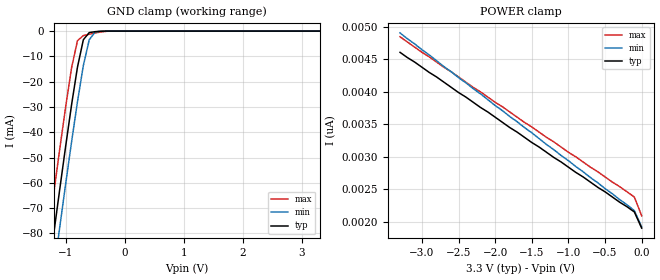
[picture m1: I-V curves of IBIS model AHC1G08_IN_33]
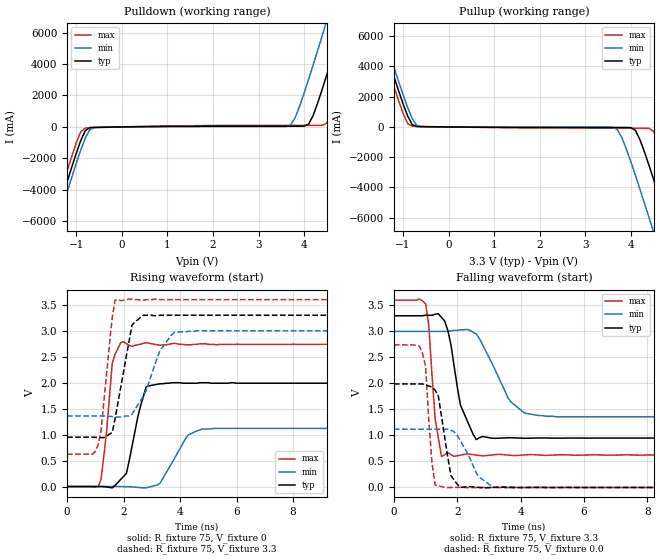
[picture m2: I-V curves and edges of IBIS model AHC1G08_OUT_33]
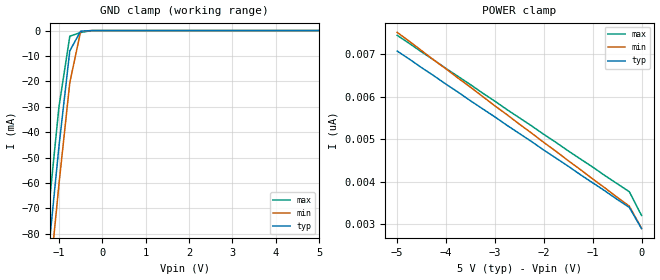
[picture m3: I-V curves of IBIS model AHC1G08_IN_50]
| TEXAS INSTRUMENTS INCORPORATED
| Standard Linear and Logic Group
| IBIS Model of SN74AHC1G08
| SINGLE 2-INPUT POSITIVE-AND GATE
| SOT 5-pin (DCK) and SOT 5-pin (DBV) Package
[IBIS Ver]   3.2
[Comment Char]  |_char
[File Name]   ahc1g08.ibs
[File Rev]   2.0 J_die
[Date]   May 24, 2000
[Source]   Data created from HSPICE simulations at TI-SLL.
[Notes]   The following is an IBIS list for the AHC1G08.
|   Please contact sllibis@ti.com with questions and
|   comments concerning SLL IBIS models.
[Disclaimer] Property of Texas Instruments Incorporated.  Unauthorized
   reproduction and/or distribution is strictly prohibited.
   This product is protected under copyright law.
   Created 2000, (C) Copyright 2000, Texas Instruments Inc.,
   All Rights Reserved.
   UNLESS THERE IS A SIGNED, WRITTEN AGREEMENT TO THE
   CONTRARY, TEXAS INSTRUMENTS () IS PROVIDING THE IBIS
   MODELS  AND WITHOUT ANY WARRANTY, EXPRESSED OR
   IMPLIED.  TI assumes no liability for:
   1) the accuracy of the IBIS models provided to your
   company;
   2) the proper functioning of these IBIS Models in your
   design or for any resulting applications; or
   3) infringement of patents, copyrights or intellectual
   property rights resulting from your use of these IBIS
   models.
   TI provides IBIS Models as a service to our customers.
   You and your company shall not distribute, sell or give
   these models to anyone else without prior written
   permission from TI.
   TI reserves the right to make changes to our products or
   to discontinue any semiconductor product or service
   without notice, and advises our customers to obtain the
   latest version of relevant information to verify, before
   placing orders, that the information being relied on is
   current.
   Please be aware that your receipt and use of the IBIS
   information provided shall serve as acceptance of these
   terms and conditions.  If you do not accept these terms,
   you should return or destroy the IBIS models and any
   other accompanying information immediately.
|   Component AHC1G08_DCK
[Component]   AHC1G08_DCK
[Manufacturer]  Texas Instruments, Inc.
[Package]
|   typ   min   max
R_pkg   0.020   0.017   0.025
L_pkg   0.998nH   0.881nH   1.069nH
C_pkg   0.146pF   0.118pF   0.205pF
[Pin]   signal_name   model_name   R_pin   L_pin   C_pin
1   A   AHC1G08_IN   0.019   1.069nH   0.162pF
2   B   AHC1G08_IN   0.018   0.881nH   0.121pF
3   GND   GND   0.017   1.031nH   0.205pF
4   Y   AHC1G08_OUT   0.020   0.960nH   0.124pF
5   VCC   POWER   0.025   1.049nH   0.118pF
|   Component AHC1G08_DBV
[Component]   AHC1G08_DBV
[Manufacturer]  Texas Instruments, Inc.
[Package]
|   typ   min   max
R_pkg   0.025   0.021   0.029
L_pkg   1.529nH   1.312nH   1.906nH
C_pkg   0.156pF   0.110pF   0.240pF
[Pin]   signal_name   model_name   R_pin   L_pin   C_pin
1   A   AHC1G08_IN   0.021   1.511nH   0.144pF
2   B   AHC1G08_IN   0.023   1.312nH   0.138pF
3   GND   GND   0.029   1.906nH   0.240pF
4   Y   AHC1G08_OUT   0.026   1.541nH   0.150pF
5   VCC   POWER   0.025   1.374nH   0.110pF
[Model Selector]   AHC1G08_IN
AHC1G08_IN_33   3.3-V Vcc Input Model
AHC1G08_IN_50   5.0-V Vcc Input Model
[Model Selector]   AHC1G08_OUT
AHC1G08_OUT_33   3.3-V Vcc Output Model
AHC1G08_OUT_50   5.0-V Vcc Output Model
| Models and submodels in the file (4): AHC1G08_IN_33 (Input), AHC1G08_OUT_33 (Output), AHC1G08_IN_50 (Input), AHC1G08_OUT_50 (Output)
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|   Model AHC1G08_IN_33
[Model]   AHC1G08_IN_33
Model_type  Input
Polarity   Inverting
Vinl = 0.99
Vinh = 2.31
| variable   typ   min   max
C_comp   1.27pf   0.95pf   1.59pf
[Temperature Range]   25   85   -40
[Voltage Range]   3.3   3.0   3.6
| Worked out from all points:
|   GND clamp passes 1 mA (typ) near -0.61 V on its own axis
[GND Clamp]
|   Voltage   I(typ)   I(min)   I(max)
-3.3V     -460mA     -475mA     -445mA
-1.3V     -97.5mA    -113mA     -81.5mA
-1.2V     -79.9mA    -95mA      -63.9mA
-1.1V     -62.6mA    -77.6mA    -46.7mA
-1V       -45.6mA    -60.5mA    -30mA
-900mV    -29.2mA    -43.9mA    -14.6mA
-800mV    -14.3mA    -28mA      -3.81mA
-700mV    -3.42mA    -13.6mA    -1.78mA
-600mV    -581uA     -3.4mA     -1.25mA
-500mV    -233uA     -353uA     -759uA
-400mV    -58.1uA    -21.9uA    -324uA
3.3V      1.9nA      2.34nA     1.69nA
[POWER Clamp]
|   Voltage   I(typ)   I(min)   I(max)
-3.3V     4.61nA     4.91nA     4.85nA
-3V       4.38nA     4.65nA     4.61nA
-100mV    2.15nA     2.17nA     2.38nA
0V        1.9nA      1.92nA     2.09nA
|   Model AHC1G08_OUT_33
[Model]   AHC1G08_OUT_33
Model_type  Output
Polarity   Inverting
Vmeas = 1.65v
Cref = 15pf
| variable   typ   min   max
C_comp   3.12pf   2.34pf   3.90pf
[Temperature Range]   25   85   -40
[Voltage Range]   3.3   3.0   3.6
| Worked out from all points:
|   slope of the pulldown table from 0 to 0.495 V, typ, clamps not added: 26.1 ohm
|   slope of the pullup table from 0 to 0.495 V, typ, clamps not added: 40.3 ohm
|   rising waveform, R_fixture 75, V_fixture 0: 20-80 % time 464ps typ, 702ps min, 278ps max; typ from 0 V to 1.99 V
|   falling waveform, R_fixture 75, V_fixture 3.3: 20-80 % time 446ps typ, 783ps min, 217ps max; typ from 3.3 V to 0.95 V
|   rising waveform, R_fixture 75, V_fixture 3.3: 20-80 % time 470ps typ, 718ps min, 323ps max; typ from 0.95 V to 3.3 V
|   falling waveform, R_fixture 75, V_fixture 0.0: 20-80 % time 308ps typ, 566ps min, 179ps max; typ from 1.99 V to 0 V
[Pulldown]
|   Voltage   I(typ)   I(min)   I(max)
-3.3V     -24A       -24.6A     -23.4A
-1.6V     -7.31A     -7.95A     -6.63A
-1.5V     -6.34A     -6.99A     -5.66A
-1V       -1.69A     -2.33A     -1.02A
-800mV    -234mA     -703mA     -70.7mA
-600mV    -28.4mA    -27.3mA    -48.1mA
3.7V      47.1mA     113mA      100mA
4.1V      173mA      3.03A      101mA
4.4V      2.42A      5.83A      105mA
4.8V      6.17A      9.67A      2.68A
5.2V      10A        13.6A      6.5A
6.6V      23.8A      27.4A      20.3A
[Pullup]
|   Voltage   I(typ)   I(min)   I(max)
-3.3V     23.8A      24.4A      23.2A
-1.6V     7.13A      7.74A      6.5A
-1.5V     6.17A      6.78A      5.53A
-1V       1.53A      2.14A      903mA
-800mV    158mA      559mA      49mA
-600mV    19.5mA     16.8mA     33.4mA
3.7V      -35.9mA    -168mA     -78.9mA
4.1V      -236mA     -3.23A     -83.5mA
4.4V      -2.58A     -6.03A     -95.5mA
4.8V      -6.34A     -9.88A     -2.81A
5.2V      -10.2A     -13.8A     -6.63A
6.6V      -24A       -27.6A     -20.4A
[Ramp]
| variable   typ   min   max
dV/dt_r   1.20E+00/4.62E-10   6.92E-01/6.38E-10   1.65E+00/2.74E-10
dV/dt_f   1.44E+00/4.29E-10   1.01E+00/7.49E-10   1.87E+00/2.29E-10
R_load = 75
[Rising Waveform]
R_fixture = 75
V_fixture = 0
|   Time   V(typ)   V(min)   V(max)
0s        0V         0V         0V
1.2ns     950uV      243uV      135mV
1.4ns     -8.38mV    656uV      1.07V
1.6ns     -25.1mV    1.08mV     2.38V
2ns       195mV      -1.74mV    2.79V
2.8ns     1.92V      -24.1mV    2.77V
3.3ns     1.98V      70.8mV     2.72V
4.3ns     1.99V      1V         2.73V
4.8ns     2V         1.11V      2.75V
25ns      1.99V      1.12V      2.74V
[Falling Waveform]
R_fixture = 75
V_fixture = 3.3
V_fixture_min = 3.0
V_fixture_max = 3.6
|   Time   V(typ)   V(min)   V(max)
0s        3.3V       3V         3.6V
1ns       3.31V      3V         3.53V
1.1ns     3.31V      3V         3.11V
1.3ns     3.33V      3V         1.32V
1.5ns     3.27V      3V         597mV
2.1ns     1.58V      3.03V      622mV
2.6ns     921mV      2.95V      623mV
3.7ns     956mV      1.64V      618mV
4.6ns     952mV      1.38V      624mV
25ns      950mV      1.36V      624mV
[Rising Waveform]
R_fixture = 75
V_fixture = 3.3
V_fixture_min = 3.0
V_fixture_max = 3.6
|   Time   V(typ)   V(min)   V(max)
0s        950mV      1.36V      624mV
1.1ns     945mV      1.36V      805mV
1.2ns     943mV      1.36V      1.06V
1.6ns     1.04V      1.35V      3.26V
1.7ns     1.31V      1.34V      3.59V
2.3ns     3.11V      1.39V      3.61V
2.7ns     3.3V       1.74V      3.59V
3.3ns     3.3V       2.63V      3.6V
3.8ns     3.3V       2.97V      3.6V
25ns      3.3V       3V         3.6V
[Falling Waveform]
R_fixture = 75
V_fixture = 0.0
|   Time   V(typ)   V(min)   V(max)
0s        1.99V      1.12V      2.74V
900ps     1.99V      1.12V      2.58V
1ns       1.97V      1.12V      2.32V
1.2ns     1.93V      1.12V      477mV
1.3ns     1.87V      1.12V      47.1mV
1.6ns     972mV      1.12V      4.07mV
1.8ns     226mV      1.1V       -193uV
2ns       60.8mV     1V         3.06mV
3.2ns     1.71mV     3.36mV     294uV
25ns      0V         0V         0V
|   Model AHC1G08_IN_50
[Model]   AHC1G08_IN_50
Model_type  Input
Polarity   Inverting
Vinl = 1.5
Vinh = 3.5
| variable   typ   min   max
C_comp   1.27pf   0.95pf   1.59pf
[Temperature Range]   25   85   -40
[Voltage Range]   5.0   4.5   5.5
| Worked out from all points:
|   GND clamp passes 1 mA (typ) near -0.52 V on its own axis
[GND Clamp]
|   Voltage   I(typ)   I(min)   I(max)
-5V       -773mA     -786mA     -758mA
-1.5V     -133mA     -148mA     -117mA
-1.25V    -88.7mA    -104mA     -72.7mA
-1V       -45.6mA    -60.5mA    -30mA
-750mV    -7.99mA    -20.5mA    -2.23mA
-500mV    -233uA     -353uA     -759uA
-250mV    -2.63nA    -182nA     -26.9uA
5V        2.9nA      3.64nA     2.54nA
[POWER Clamp]
|   Voltage   I(typ)   I(min)   I(max)
-5V       7.08nA     7.52nA     7.45nA
-1.5V     4.37nA     4.5nA      4.73nA
-250mV    3.4nA      3.43nA     3.77nA
0V        2.9nA      2.91nA     3.21nA
